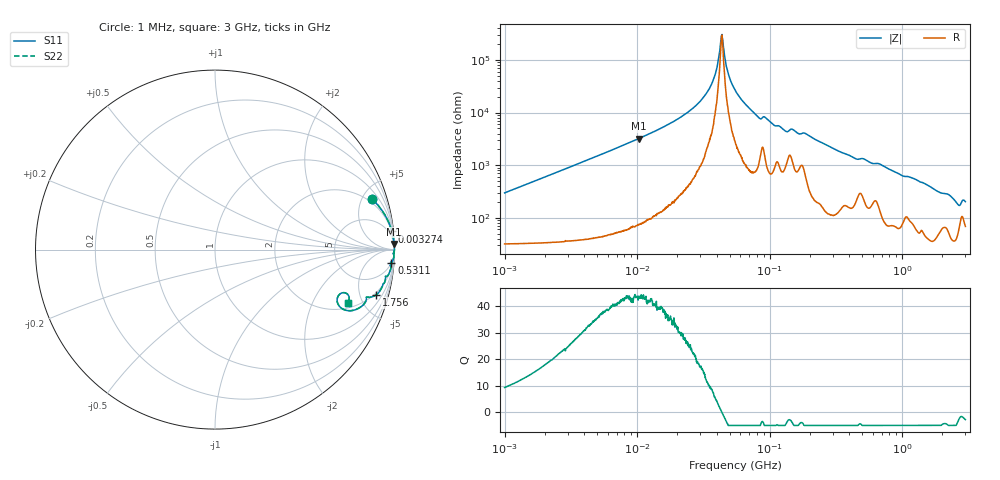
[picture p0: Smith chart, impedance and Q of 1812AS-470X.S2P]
!s-Parameter Generated by FASTRON Sdn. Bhd.
!FASTRON P/N : 1812AS-470X
!Keysight Technologies,E4991B,MY54100416,A.01.15
!Date created: Mon Oct 16 10:12:16 2023
!Version  : Mon Oct 16 10:12:16 2023
!Data & Calibration Information:
!Freq	S11	S21	S12	S22
!PortZ  Port1:50+j0  Port2:50+j0
!When reading, reference impedance value at option line is always used.
! Remarks : This data is being provided solely for informational purposes.
# Hz S dB R 50
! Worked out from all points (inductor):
!   1601 points, 1 MHz to 3 GHz, reference 50 ohm
!   read as one part in series: L = 47 uH near 1.041 MHz
!   highest Q = 43.6 at 10.3 MHz (marker M1), where L = 49.5 uH
!   self-resonance near 43.51 MHz
!   S11 on the Smith chart (normalised r, x): 1 MHz: 1.64, +5.91; 3.274 MHz: 2, +19; 531.1 MHz: 4, -25; 1.756 GHz: 1.75, -6.85; 3 GHz: 2.37, -3.81
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1000000  -0.74 17.9  -10.20 -66.0  -10.20 -66.0  -0.74 17.9
3273773  -0.08 5.9  -19.82 -82.0  -19.82 -82.0  -0.08 5.9
3804036  -0.06 5.0  -21.12 -83.0  -21.12 -83.0  -0.06 5.0
1.029702e7  -0.01 1.8  -30.12 -86.9  -30.12 -86.9  -0.01 1.8
1.447069e7  -0.01 1.2  -33.57 -87.3  -33.57 -87.3  -0.01 1.2
2.386763e7  -0.00 0.6  -39.95 -87.2  -39.95 -87.2  -0.00 0.6
3.238729e7  -0.00 0.3  -46.42 -85.7  -46.42 -85.7  -0.00 0.3
3.820236e7  -0.00 0.1  -53.43 -80.4  -53.43 -80.4  -0.00 0.1
4.351043e7  -0.00 0.0  -69.29 -3.3  -69.29 -3.3  -0.00 0.0
4.461279e7  -0.00 -0.0  -65.91 48.1  -65.91 48.1  -0.00 -0.0
4.881767e7  -0.00 -0.1  -54.59 78.8  -54.59 78.8  -0.00 -0.1
5.477226e7  -0.00 -0.2  -48.60 83.7  -48.60 83.7  -0.00 -0.2
8.338914e7  -0.02 -0.7  -37.93 81.0  -37.93 81.0  -0.02 -0.7
9.262894e7  -0.02 -0.7  -38.19 80.0  -38.19 80.0  -0.02 -0.7
1.321429e8  -0.04 -1.3  -32.96 76.4  -32.96 76.4  -0.04 -1.3
1.482612e8  -0.05 -1.1  -33.71 74.7  -33.71 74.7  -0.05 -1.1
2.083556e8  -0.02 -1.7  -30.52 83.9  -30.52 83.9  -0.02 -1.7
5.311214e8  -0.12 -4.4  -22.14 77.6  -22.14 77.6  -0.12 -4.4
7.925923e8  -0.14 -6.7  -18.69 78.6  -18.69 78.6  -0.14 -6.7
1.75626e9  -0.60 -15.6  -11.34 68.1  -11.34 68.1  -0.60 -15.6
2.607784e9  -1.91 -24.9  -7.26 51.1  -7.26 51.1  -1.91 -24.9
3e9  -1.98 -21.7  -8.10 48.5  -8.10 48.5  -1.98 -21.7
